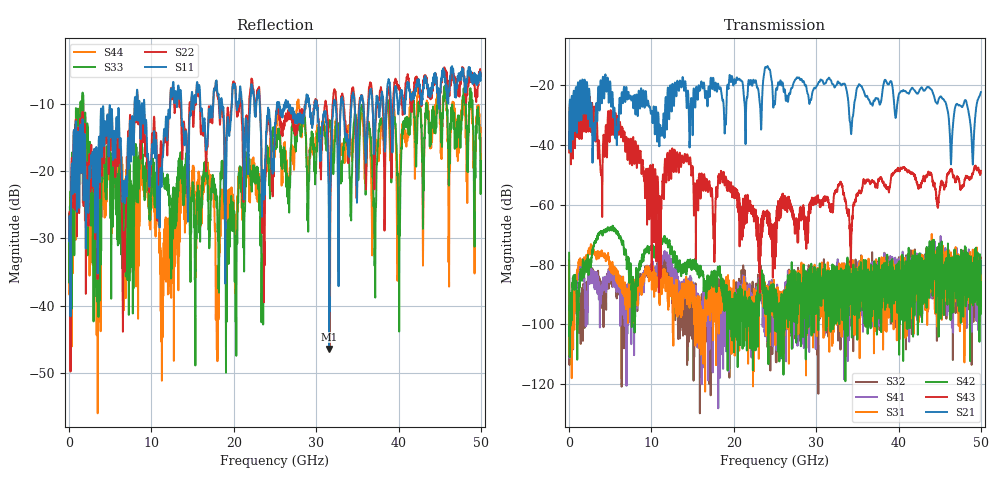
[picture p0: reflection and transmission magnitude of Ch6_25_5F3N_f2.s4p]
!Agilent Technologies,N5247A,US51170199,A.09.90.13
!Agilent N5247A: A.09.90.13
!Date: Wednesday, December 16, 2015 09:57:03
!Correction: S11(Full 4 Port(1,2,3,4))
!S12(Full 4 Port(1,2,3,4))
!S13(Full 4 Port(1,2,3,4))
!S14(Full 4 Port(1,2,3,4))
!S21(Full 4 Port(1,2,3,4))
!S22(Full 4 Port(1,2,3,4))
!S23(Full 4 Port(1,2,3,4))
!S24(Full 4 Port(1,2,3,4))
!S31(Full 4 Port(1,2,3,4))
!S32(Full 4 Port(1,2,3,4))
!S33(Full 4 Port(1,2,3,4))
!S34(Full 4 Port(1,2,3,4))
!S41(Full 4 Port(1,2,3,4))
!S42(Full 4 Port(1,2,3,4))
!S43(Full 4 Port(1,2,3,4))
!S44(Full 4 Port(1,2,3,4))
!S4P File: Measurements: <S11,S12,S13,S14>,
!<S21,S22,S23,S24>,
!<S31,S32,S33,S34>,
!<S41,S42,S43,S44>:
# Hz S  dB  R 50
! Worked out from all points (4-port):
!   3201 points, 10 MHz to 50 GHz, reference 50 ohm
!   strongest paths, dB at 10 MHz, 12.51 GHz, 25 GHz, 37.5 GHz, 50 GHz:
!     S21: -41.2, -21.6, -26.3, -24.5, -22.4
!     S43: -42.5, -42.0, -81.3, -52.6, -48.7
!     S42: -76.0, -75.2, -90.9, -89.8, -86.4
!     S31: -78.6, -86.2, -103.4, -87.3, -86.0
!     S41: -79.9, -80.4, -106.3, -79.9, -78.4
!     S32: -84.8, -86.5, -95.1, -84.7, -82.9
!   lowest |S11| = -46.4 dB at 31.58 GHz (marker M1), VSWR 1.01, Z = 49.6 - j0.188 ohm
!   |S11| at or under -10 dB: start of sweep to 7.959 GHz; 9.143 GHz to 12.29 GHz (3.142 GHz wide, 29.3 % of centre); 23.13 GHz to 25.24 GHz (2.108 GHz wide, 8.72 % of centre)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
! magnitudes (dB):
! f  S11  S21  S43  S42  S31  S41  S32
! 10 MHz  -30.4  -41.2  -42.5  -76.0  -78.6  -79.9  -84.8
! 5.774 GHz  -12.0  -38.0  -36.7  -69.3  -83.5  -89.2  -86.6
! 11.05 GHz  -22.9  -33.5  -58.6  -73.4  -87.2  -78.7  -84.6
! 12.54 GHz  -8.5  -19.9  -41.1  -76.1  -89.7  -81.9  -87.0
! 23.08 GHz  -8.2  -24.0  -82.5  -89.5  -85.7  -93.0  -86.4
! 31.58 GHz  -46.4  -17.6  -61.1  -88.3  -88.9  -90.4  -85.2
! 50 GHz  -5.6  -22.4  -48.7  -86.4  -86.0  -78.4  -82.9
